// generates a signal build up by the specified function type. v1.6
FUNCTION_BLOCK FB_FunctionGenerator
VAR_INPUT
	bEnable				: BOOL 	:= TRUE;		// set TRUE to generate the specified signal; set FALSE to reset the signal buffer
	fFrequency			: LREAL := 1000;		// signal frequency [Hz]
	fAmplitude			: LREAL := 1;			// signal amplitude [V]
	fOffset				: LREAL	:= 0;	
	nDutyCycle			: UINT 	:= 50;			// change in percent of period [%] (for pulse/shock function)
	eFunction			: E_FunctionType := E_FunctionType.Sine;
	fSampleRate			: LREAL := 0.0;			// samplerate for user scaling [Hz] default: disabled
	fCarrierFrequency	: LREAL := 500;			// carrier frequency [Hz]
	fCarrierAmplitude	: LREAL := 1.0;			// carrier amplitude [V] default: disabled
END_VAR
VAR_IN_OUT
	aSignal		: ARRAY[1..cOversamples] OF LREAL;
END_VAR
VAR_OUTPUT
	bError		: BOOL;
END_VAR

VAR
	bInit						: BOOL := TRUE;
	fbGetTaskIdx				: GETCURTASKINDEX;
	
	fLastFrequency				: LREAL;		// in [Hz]
	fLastAmplitude				: LREAL;
	fLastOffset					: LREAL;
	nLastDutyCycle				: UINT;
	eLastFunction				: E_FunctionType;
	
	nSamples					: UDINT;
	fCycleTime					: LREAL;		// in [s]
	fDelta						: LREAL;		// amplitude delta per sample
	fPhase						: LREAL;		// in [°]
	nSign						: INT := 1;		// 1 or -1
	fLastSignalValue			: LREAL;		// amplitude
	fPeriod						: LREAL;		// in [s]
	fAngularIncrement			: LREAL;		// in [°]
	fAngularIncrementPerCycle	: LREAL;		// in [°]
	fAngularIncrementPerSample	: LREAL;		// in [°]
	(* for modulated signal (carrier signal without offset) *)
	fCarrierPeriod						: LREAL;		// in [s]
	fCarrierAngularIncrement			: LREAL;		// in [°]
	fCarrierAngularIncrementPerCycle	: LREAL;		// in [°]
	fCarrierAngularIncrementPerSample	: LREAL;		// in [°]
	(* for harmonic tone complex *)
	h							: UDINT;	
	nHarmonics					: UDINT := 5;
END_VAR

IF bEnable THEN
	IF fLastFrequency <> fFrequency THEN
		bInit := TRUE; // For automatic initializing
		fLastFrequency := fFrequency;
	END_IF
	IF fLastAmplitude <> fAmplitude THEN
		bInit := TRUE; // For automatic initializing
		fLastAmplitude := fAmplitude;
	END_IF
	IF fLastOffset <> fOffset THEN
		bInit := TRUE; // For automatic initializing
		fLastOffset := fOffset;
	END_IF
	IF nLastDutyCycle <> nDutyCycle THEN
		bInit := TRUE; // For automatic initializing
		nLastDutyCycle := nDutyCycle;
	END_IF
	IF eLastFunction <> eFunction THEN
		bInit := TRUE; // For automatic initializing
		eLastFunction := eFunction;
	END_IF
	IF bInit THEN
		// Get task info	
		fbGetTaskIdx();
		fCycleTime := UDINT_TO_LREAL(TwinCAT_SystemInfoVarList._TaskInfo[fbGetTaskIdx.index].CycleTime);	// [100ns]
		fCycleTime := fCycleTime / (10.0 * 1000.0 * 1000.0);												// [s]
		// Override samplerate
		IF fSampleRate > 0.0 THEN
			fCycleTime := fCycleTime * fSampleRate / UDINT_TO_LREAL(TwinCAT_SystemInfoVarList._TaskInfo[fbGetTaskIdx.index].CycleTime);
		END_IF
		
		fLastSignalValue := 0;
		nSign := 1;
		fAngularIncrement := 0;
		// Flush out old data
		MEMSET(ADR(aSignal), 0, SIZEOF(aSignal));
		IF fFrequency > 0 AND fCycleTime > 0 THEN		
			// Calculate period, increments per plc cycle, increment per oversample
			IF cOversamples > 0 THEN			
				IF eFunction = E_FunctionType.Sine THEN
					fPeriod := 1/fFrequency;
					fAngularIncrementPerCycle := 360*(fCycleTime/fPeriod);
					fAngularIncrementPerSample := fAngularIncrementPerCycle/cOversamples;
					// no phase adjustment
					bInit := FALSE;	
				ELSIF eFunction = E_FunctionType.Square	THEN
					fPeriod := 1/fFrequency;
					fAngularIncrementPerCycle  := 360*(fCycleTime/fPeriod);
					fAngularIncrementPerSample := fAngularIncrementPerCycle/cOversamples;
					fPhase := 0.5*360;
					bInit := FALSE;
				ELSIF eFunction = E_FunctionType.Pulse THEN
					fPeriod := 1/fFrequency;
					fAngularIncrementPerCycle  := 360*(fCycleTime/fPeriod);
					fAngularIncrementPerSample := fAngularIncrementPerCycle/cOversamples;
					IF nDutyCycle > 100 THEN
						nDutyCycle := 100;
					END_IF
					fPhase := (UDINT_TO_LREAL(nDutyCycle)/100)*360;
					bInit := FALSE;					
				ELSIF eFunction = E_FunctionType.Triangular THEN
					fPeriod := 1/fFrequency;				
					fAngularIncrementPerCycle  := 360*(fCycleTime/fPeriod);
					fAngularIncrementPerSample := fAngularIncrementPerCycle/cOversamples;
					fPhase := 0.5*360; 
					fDelta := 4*(fAmplitude/(360/fAngularIncrementPerSample));				
					bInit := FALSE;
				ELSIF eFunction = E_FunctionType.Sawtooth THEN
					fPeriod := 1/fFrequency;			
					fAngularIncrementPerCycle  := 360*(fCycleTime/fPeriod);		
					fAngularIncrementPerSample := fAngularIncrementPerCycle/cOversamples;
					fDelta := fAmplitude/(360/fAngularIncrementPerSample);
					bInit := FALSE;
				ELSIF eFunction = E_FunctionType.AM THEN
					fPeriod := 1/fFrequency;
					fAngularIncrementPerCycle := 360*(fCycleTime/fPeriod);
					fAngularIncrementPerSample := fAngularIncrementPerCycle/cOversamples;
					// no phase adjustment
					fCarrierPeriod := 1/fCarrierFrequency;
					fCarrierAngularIncrementPerCycle := 360*(fCycleTime/fCarrierPeriod);
					fCarrierAngularIncrementPerSample := fCarrierAngularIncrementPerCycle/cOversamples;				
					// no phase adjustment	
					bInit := FALSE;
				ELSIF eFunction = E_FunctionType.Harmonics THEN
					fPeriod := 1/fFrequency;
					fAngularIncrementPerCycle := 360*(fCycleTime/fPeriod);
					fAngularIncrementPerSample := fAngularIncrementPerCycle/cOversamples;
					// no phase adjustment
					bInit := FALSE;
				ELSIF eFunction = E_FunctionType.Shock THEN
					fPeriod := 1/fFrequency;			
					fAngularIncrementPerCycle  := 360*(fCycleTime/fPeriod);		
					fAngularIncrementPerSample := fAngularIncrementPerCycle/cOversamples;
					IF nDutyCycle > 100 THEN
						nDutyCycle := 100;
					END_IF
					fLastSignalValue := fAmplitude;
					bInit := FALSE;	
				ELSIF eFunction = E_FunctionType.Shockwave THEN
					// carrier
					fCarrierPeriod := 1/fCarrierFrequency;
					fCarrierAngularIncrementPerCycle := 360*(fCycleTime/fCarrierPeriod);
					fCarrierAngularIncrementPerSample := fCarrierAngularIncrementPerCycle/cOversamples;
					// shock
					fPeriod := 1/fFrequency;			
					fAngularIncrementPerCycle  := 360*(fCycleTime/fPeriod);		
					fAngularIncrementPerSample := fAngularIncrementPerCycle/cOversamples;
					IF nDutyCycle > 100 THEN
						nDutyCycle := 100;
					END_IF
					fLastSignalValue := fAmplitude;
					bInit := FALSE;	
				ELSE
					bError := TRUE;	
				END_IF
			ELSE
				bError := TRUE;
			END_IF
		ELSE
			bError := TRUE;
		END_IF
	END_IF
	
	// Enable function generator
	IF NOT bError THEN		
		CASE eFunction OF		
			// sine: typical for vibrations originating from rotating machine
			E_FunctionType.Sine: Sine();
			
			// square: mixed sine signals good for analyzing spectrum				
			E_FunctionType.Square: Square();
			
			// pulse: mixed sine signals good for analyzing spectrum				
			E_FunctionType.Pulse: Pulse();
	
			// sawtooth: ramp-type vibrations, continuously increasing			
			E_FunctionType.Sawtooth: Sawtooth();
		
			// triangular: mixed sine signals good for analyzing spectrum
			E_FunctionType.Triangular: Triangular();
		
			// amplitude modulation: typical for vibrations originating from gear-tooth failure or bearing faults
			// Carrier signal with own frequency and amplitude		
			E_FunctionType.AM: AM();
			
			// harmonic tone complex
			E_FunctionType.Harmonics: Harmonics();

			// shock with exponential decay
			E_FunctionType.Shock: Shock();
			
			// shockwave with exponential decay
			E_FunctionType.Shockwave: Shockwave();
		END_CASE
	END_IF
ELSE
	// Flush out old data
	MEMSET(ADR(aSignal), 0, SIZEOF(aSignal));
	
	bInit := TRUE;
	bError := FALSE;
END_IF

METHOD PRIVATE AM
VAR_INPUT
END_VAR
{warning disable C0371}

FOR nSamples := 1 TO cOversamples DO
	// base signal * carrier signal
	aSignal[nSamples] := ( fAmplitude*SIN(2*PI*(fAngularIncrement+(nSamples-1)*fAngularIncrementPerSample)/360) + fOffset )
							* ( fCarrierAmplitude*SIN(2*PI*(fCarrierAngularIncrement+(nSamples-1)*fCarrierAngularIncrementPerSample)/360) );
END_FOR
// Increment angular positions
fAngularIncrement := fAngularIncrement + fAngularIncrementPerCycle;
fCarrierAngularIncrement := fCarrierAngularIncrement + fCarrierAngularIncrementPerCycle;

{warning restore C0371}
END_METHOD

METHOD PRIVATE Harmonics
VAR_INPUT
END_VAR
VAR
	
	
END_VAR
{warning disable C0371}

FOR nSamples := 1 TO cOversamples DO
	aSignal[nSamples] := 0;
	FOR h := 1 TO nHarmonics DO
		aSignal[nSamples] := aSignal[nSamples] +  fAmplitude*SIN(2*PI*h*(fAngularIncrement+(nSamples-1)*fAngularIncrementPerSample)/360);
	END_FOR
	aSignal[nSamples] := aSignal[nSamples] + fOffset;
END_FOR

// Increment angular position
fAngularIncrement := fAngularIncrement + fAngularIncrementPerCycle;

{warning restore C0371}
END_METHOD

METHOD PRIVATE Pulse
VAR_INPUT
END_VAR
{warning disable C0371}

FOR nSamples := 1 TO cOversamples DO
	// For pulse wave (unequal phases)
	IF (fAngularIncrement >= 360) THEN
		fAngularIncrement := fAngularIncrement - DINT_TO_LREAL(LREAL_TO_DINT(fAngularIncrement/360))*360;
		// or with Tc2_Math library: fAngularIncrement := LMOD(fAngularIncrement,360);
	END_IF
	IF (fAngularIncrement < fPhase) THEN
		nSign := 1;		
	ELSIF (fAngularIncrement >= fPhase) THEN
		nSign := 0;
	END_IF
	fAngularIncrement := fAngularIncrement + fAngularIncrementPerSample;
	
	aSignal[nSamples] := nSign*fAmplitude;
	
	aSignal[nSamples] := aSignal[nSamples] + fOffset;
END_FOR

{warning restore C0371}
END_METHOD

METHOD PRIVATE Sawtooth
VAR_INPUT
END_VAR
{warning disable C0371}

FOR nSamples := 1 TO cOversamples DO
	// For sawtooth wave (equal phase = period/2)
	IF (fAngularIncrement >= 360) THEN
		fAngularIncrement := fAngularIncrement - DINT_TO_LREAL(LREAL_TO_DINT(fAngularIncrement/360))*360;
		// or with Tc2_Math library: fAngularIncrement := LMOD(fAngularIncrement,360);
		fLastSignalValue := fLastSignalValue -fAmplitude;
	END_IF
	fAngularIncrement := fAngularIncrement + fAngularIncrementPerSample;

	aSignal[nSamples] := fLastSignalValue + fDelta;

	// Store last sample
	fLastSignalValue := aSignal[nSamples];
	
	aSignal[nSamples] := aSignal[nSamples] + fOffset;					
END_FOR	

{warning restore C0371}
END_METHOD

METHOD PRIVATE Shock
VAR
	tol		: LREAL := 1E-4;
	lambda	: LREAL := LOG(tol) / MIN((UINT_TO_LREAL(nDutyCycle)/100), 1);
END_VAR
VAR_INPUT
END_VAR
{warning disable C0371}

FOR nSamples := 1 TO cOversamples DO
	// For sawtooth wave (equal phase = period/2)
	IF (fAngularIncrement >= 360) THEN
		fAngularIncrement := fAngularIncrement - DINT_TO_LREAL(LREAL_TO_DINT(fAngularIncrement/360))*360;
		// or with Tc2_Math library: fAngularIncrement := LMOD(fAngularIncrement,360);
	END_IF
	aSignal[nSamples] := fAmplitude * EXP( lambda * ((fAngularIncrement)/360) );
	fAngularIncrement := fAngularIncrement + fAngularIncrementPerSample;
	// Store last sample
	fLastSignalValue := aSignal[nSamples];
	aSignal[nSamples] := aSignal[nSamples] + fOffset;					
END_FOR	

{warning restore C0371}
END_METHOD

METHOD Shockwave : BOOL
VAR
	tol		: LREAL := 1E-4;
	lambda	: LREAL := LOG(tol) / MIN((UINT_TO_LREAL(nDutyCycle)/100), 1);
END_VAR
VAR_INPUT
END_VAR
{warning disable C0371}

FOR nSamples := 1 TO cOversamples DO
	// For shock wave exponential decay
	IF (fCarrierAngularIncrement >= 360) THEN
		fCarrierAngularIncrement := fCarrierAngularIncrement - DINT_TO_LREAL(LREAL_TO_DINT(fCarrierAngularIncrement/360))*360;
		fAngularIncrement := fAngularIncrement - DINT_TO_LREAL(LREAL_TO_DINT(fAngularIncrement/360))*360;
	END_IF
	// exponential decay
	aSignal[nSamples] := fCarrierAmplitude*EXP(lambda*((fCarrierAngularIncrement)/360));
	fCarrierAngularIncrement := fCarrierAngularIncrement + fCarrierAngularIncrementPerSample;
	// multiply with sine wave
	aSignal[nSamples] := aSignal[nSamples] * fAmplitude * COS(2*PI*(fAngularIncrement+(nSamples-1)*fAngularIncrementPerSample)/360);
	// Store last sample
	fLastSignalValue := aSignal[nSamples];
	// add offset
	aSignal[nSamples] := aSignal[nSamples] + fOffset;		
END_FOR	
fAngularIncrement := fAngularIncrement + fAngularIncrementPerCycle;

{warning restore C0371}
END_METHOD

METHOD PRIVATE Sine
VAR_INPUT
END_VAR
{warning disable C0371}

FOR nSamples := 1 TO cOversamples DO
	aSignal[nSamples] := fAmplitude*SIN(2*PI*(fAngularIncrement+(nSamples-1)*fAngularIncrementPerSample)/360);

	aSignal[nSamples] := aSignal[nSamples] + fOffset;
END_FOR

// Increment angular position
fAngularIncrement := fAngularIncrement + fAngularIncrementPerCycle;

{warning restore C0371}
END_METHOD

METHOD PRIVATE Square
VAR_INPUT
END_VAR
{warning disable C0371}

FOR nSamples := 1 TO cOversamples DO
	// For square wave (equal phase = period/2)
	IF (fAngularIncrement >= 360) THEN
		fAngularIncrement := fAngularIncrement - DINT_TO_LREAL(LREAL_TO_DINT(fAngularIncrement/360))*360;
		// or with Tc2_Math library: fAngularIncrement := LMOD(fAngularIncrement,360);
	END_IF
	IF (fAngularIncrement < fPhase) THEN
		nSign := 1;
	ELSIF (fAngularIncrement >= fPhase) THEN
		nSign := -1;
	END_IF
	fAngularIncrement := fAngularIncrement + fAngularIncrementPerSample;
	
	aSignal[nSamples] := nSign*fAmplitude;
	
	aSignal[nSamples] := aSignal[nSamples] + fOffset;
END_FOR

{warning restore C0371}
END_METHOD

METHOD PRIVATE Triangular
VAR_INPUT
END_VAR
{warning disable C0371}

FOR nSamples := 1 TO cOversamples DO
	IF (fAngularIncrement >= 360) THEN
		fAngularIncrement := fAngularIncrement - DINT_TO_LREAL(LREAL_TO_DINT(fAngularIncrement/360))*360;
		// or with Tc2_Math library: fAngularIncrement := LMOD(fAngularIncrement,360);
	END_IF
	// Negative delta -> Positive delta
	IF fAngularIncrement < fPhase/2 THEN	
		nSign := 1;		
	ELSIF fAngularIncrement >= fPhase/2 AND fAngularIncrement < 3*fPhase/2 THEN
		nSign := -1;
	ELSIF fAngularIncrement >= 3*fPhase/2 THEN
		nSign := 1;	
	END_IF
	fAngularIncrement := fAngularIncrement + fAngularIncrementPerSample;
	
	aSignal[nSamples] := fLastSignalValue + nSign*fDelta;
	IF aSignal[nSamples] > fAmplitude THEN
		aSignal[nSamples] := aSignal[nSamples] - 2*(aSignal[nSamples]-fAmplitude);
	ELSIF aSignal[nSamples] < (-1)*fAmplitude THEN
		aSignal[nSamples] := aSignal[nSamples] - 2*(aSignal[nSamples]+fAmplitude);
	END_IF
	
	// Store last sample
	fLastSignalValue := aSignal[nSamples];		
	
	aSignal[nSamples] := aSignal[nSamples] + fOffset;
END_FOR

{warning restore C0371}
END_METHOD

END_FUNCTION_BLOCK
